FUNCTION_BLOCK FB_SmoothCam
VAR_INPUT
	Execute  :BOOL;
	CamTableID : MC_CAM_ID; 
	CamTableIDAcc   : MC_CAM_ID; 
END_VAR

VAR_OUTPUT
	Done  :BOOL;
	Busy  :BOOL;
	Error  :BOOL;
	ErrorID  :UDINT;
END_VAR

VAR_IN_OUT
	Master  :axis_ref;
	Slave  :axis_ref;
END_VAR

VAR	
	mcCamIn_V2: MC_CamIn_V2;
	mcCamExchange: MC_CamExchange;
	mcCamExchange1: MC_CamExchange;
	rTRIG: R_TRIG;
	State  :INT;

	mcCamInfo: MC_CamInfo;
	MasterMemPos: LREAL;
	Switch: BOOL;
END_VAR

mcCamIn_V2(
	Master:=Master , 
	Slave:=Slave , 
	Execute:= , 
	ActivationMode:= , 
	ActivationPosition:= , 
	CamTableID:=CamTableIDAcc , 
	Scaling:= , 
	Options:= , 
	InSync=> , 
	Busy=> , 
	Active=> , 
	CommandAborted=> , 
	Error=> , 
	ErrorID=> );

mcCamExchange(
	Master:=Master , 
	Slave:=Slave , 
	Execute:= , 
	ActivationMode:= , 
	ActivationPosition:= , 
	CamTableID:= CamTableID, 
	ReferenceCamTableID:= , 
	Scaling:= , 
	Options:= , 
	InSync=> , 
	Busy=> , 
	Active=> , 
	CommandAborted=> , 
	Error=> , 
	ErrorID=> );
	
mcCamExchange1(
	Master:=Master , 
	Slave:=Slave , 
	Execute:= , 
	ActivationMode:= , 
	ActivationPosition:= , 
	CamTableID:= , 
	ReferenceCamTableID:= , 
	Scaling:= , 
	Options:= , 
	InSync=> , 
	Busy=> , 
	Active=> , 
	CommandAborted=> , 
	Error=> , 
	ErrorID=> );
	
mcCamInfo(
	Slave:=Slave , 
	Execute:= , 
	AtMasterPosition:= , 
	MasterPosition:= , 
	Done=> , 
	Busy=> , 
	Error=> , 
	ErrorID=> , 
	CamInfo=> );

	
rTRIG(CLK:=Execute , Q=> );
CASE State OF
	0:
		IF NOT Execute THEN
			Done :=FALSE;
			Busy  :=FALSE;
			Error :=FALSE;
			ErrorID  :=0;
		END_IF
		
		IF  rTRIG.Q THEN
			State:=10;
			Busy:=TRUE;
			Ini_SubFb();
		END_IF
		
	10:
		mcCamIn_V2.Execute:=TRUE;                            //使用相对模式下0~100的4号凸轮表启动凸轮表
		IF  mcCamIn_V2.InSync THEN
			State:=20;
			MasterMemPos:=Master.NcToPlc.SetPos;
		END_IF
	20:                                                       //启动后根据主轴位置计算下个周期从轴的耦合位置
		mcCamInfo.Execute:=TRUE;
		IF  mcCamInfo.Done THEN
			State:=30;
		END_IF
	30:	                                                      //下个周期开始过度为凸轮表3周期性耦合
		mcCamExchange.ActivationPosition:=-mcCamInfo.CamInfo.MasterAxisCouplingPos+100;
		mcCamExchange.Execute:=TRUE;
		State:=40;
	40:	
	
	(*使用camexchange切换非周期凸轮和周期性凸轮进行拼接使用有以下几个优点：
	1,周期性凸轮起点和终点速度不一致会导致凸轮表无法使用.
	2,对应带有速度的从轴进行耦合，可以先使用非周期耦合作为加速凸轮过度。*)
	
	
	
	
(*	
		IF Switch THEN
			mcCamExchange1.Scaling.MasterRelative:=TRUE;
			mcCamExchange1.Scaling.SlaveRelative:=TRUE;
			(*mcCamExchange.ActivationMode:=MC_CAMACTIVATION_NEXTCYCLE;*)
			mcCamExchange1.ActivationMode:=MC_CAMACTIVATION_NEXTCYCLE;
			mcCamExchange1.CamTableID:=5;
			mcCamExchange1.Execute:=TRUE;
		END_IF
*)
END_CASE

METHOD Ini_SubFb : BOOL
VAR_INPUT
END_VAR
mcCamExchange.Execute:=FALSE;
mcCamIn_V2.Execute:=FALSE;
mcCamIn_V2.Scaling.MasterRelative:=TRUE;
mcCamIn_V2.Scaling.SlaveRelative:=TRUE;
mcCamIn_V2.ActivationMode:=MC_CAMACTIVATION_INSTANTANEOUS;

mcCamExchange.Scaling.MasterRelative:=TRUE;
mcCamExchange.Scaling.SlaveRelative:=TRUE;
(*mcCamExchange.ActivationMode:=MC_CAMACTIVATION_NEXTCYCLE;*)
mcCamExchange.ActivationMode:=MC_CAMACTIVATION_ATMASTERAXISPOS;
(*mcCamExchange.Scaling.MasterScalingMode:=MC_CAMSCALING_AUTOOFFSET;*)
END_METHOD

END_FUNCTION_BLOCK
